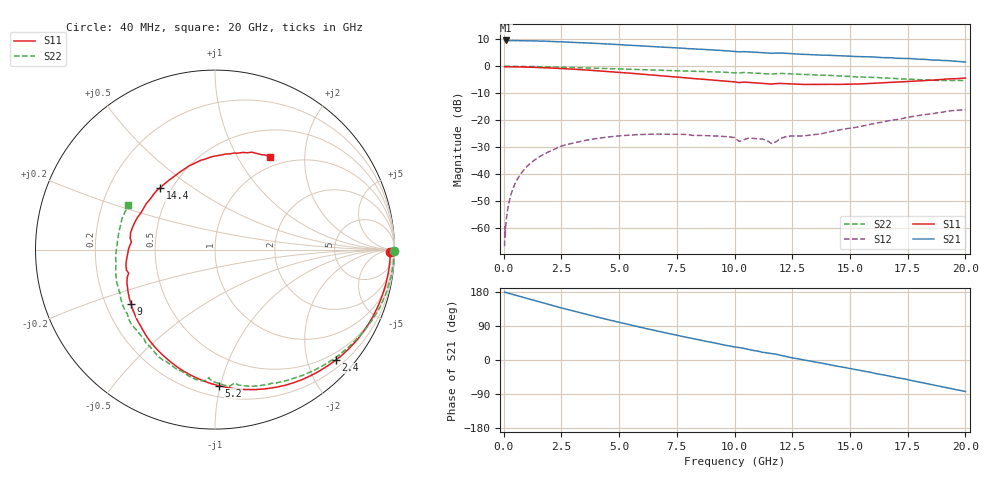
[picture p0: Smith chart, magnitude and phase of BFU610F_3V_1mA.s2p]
! Filename:  P:\Prog\Test\Noise\ATS_data\Testdata_Net\SplitFiles\BFU610_2W_A5_HighFreq_3V_1mA_D.s2p
! Date/Time: Wed 10/Aug/2011 16:56:46
! BFU610_2W_A5_HighFreq_3V_1mA_10mA_Bias1_R.s2p
! MDIF S-parameter v. bias file
! BFU610_2W_A5_HighFreq_3V_1mA_10mA
! Date/time Mon Aug 08 14:07:26 2011
! bias mode 1
! bias variable = I_out
! VAR bias_var= 1
! VAR V_out= 3.0000
! VAR I_out= 0.9950
! VAR V_in= 0.8465
! VAR I_in= 0.0072
! Device data file deembeded for feedlines and parallel
! Original file: \SplitFiles\BFU610_2W_A5_HighFreq_3V_1mA_R.s2p
! Feed-files: PR003V01_101208_Feed1.s2p, PR003V01_101208_Feed2.s2p
! Parallel-file: PR003V01_101208_Par.s2p
# MHz S MA R 50
!  Freq-MHz  S11-mag  S11-arg  S21-mag  S21-arg  S12-mag  S12-arg  S22-mag  S22-arg
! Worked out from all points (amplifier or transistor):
!   167 points, 40 MHz to 20 GHz, reference 50 ohm
!   highest |S21| = 9.6 dB at 80 MHz (marker M1)
!   |S21| within 3 dB of that: start of sweep to 7.93 GHz
!   unconditionally stable (mu >= 1): 7.857 GHz to end of sweep
!   at 550 MHz: K = -0.01, MSG = 26.0 dB, |S12| = -42.5 dB
!   at 4.2 GHz: K = 0.40, MSG = 17.5 dB, |S12| = -26.6 dB
!   at 20 GHz: K = 1.09, MAG = 6.9 dB, |S12| = -16.1 dB
!   S11 on the Smith chart (normalised r, x): 40 MHz: 68, -36; 2.4 GHz: 0.35, -2.53; 5.2 GHz: 0.28, -0.99; 9 GHz: 0.31, -0.27; 14.4 GHz: 0.43, +0.38; 20 GHz: 0.85, +1.39
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40  0.9774 -0.7  3.006 179.1  0.0004602 90.8  0.9978 -0.4
50  0.9772 -0.9  2.99 179.2  0.001057 68.9  0.9982 -0.5
60  0.9774 -1.0  2.999 178.4  0.0006629 76.0  0.9984 -0.6
80  0.9773 -1.4  3.008 178.3  0.0009905 90.2  0.9984 -0.8
140  0.9769 -2.5  2.992 177.4  0.001772 91.6  0.9982 -1.4
280  0.9756 -5.0  2.99 174.9  0.003684 90.5  0.9978 -2.7
700  0.9696 -12.6  2.971 167.7  0.009554 84.1  0.9941 -6.8
1350  0.9532 -24.1  2.956 156.5  0.01839 74.6  0.9851 -13.1
2400  0.9119 -42.5  2.842 139.1  0.03194 61.0  0.9627 -22.9
3400  0.8619 -59.3  2.724 123.3  0.04098 48.5  0.9368 -31.6
4300  0.8113 -74.0  2.616 109.7  0.04743 38.8  0.9117 -39.0
5200  0.7583 -88.4  2.486 96.7  0.05196 30.0  0.8861 -46.1
6800  0.6659 -113.5  2.274 74.5  0.05502 16.4  0.8426 -58.2
9000  0.5571 -147.1  2.011 46.6  0.05122 5.9  0.7903 -74.3
10200  0.4984 -164.7  1.848 32.9  0.04036 -0.6  0.751 -81.7
11600  0.4673 174.9  1.737 16.9  0.03685 8.9  0.7132 -92.8
12000  0.4796 168.6  1.757 12.3  0.04614 23.6  0.7354 -96.0
13400  0.4604 146.2  1.631 -4.2  0.05391 21.9  0.6921 -109.7
14400  0.4603 131.6  1.573 -15.9  0.06388 25.0  0.6654 -120.1
16800  0.5043 98.9  1.439 -43.6  0.09967 18.6  0.5994 -149.5
18400  0.5481 79.0  1.325 -63.3  0.1293 6.5  0.5552 -175.4
20000  0.6034 59.2  1.198 -83.2  0.1571 -9.9  0.5437 152.9
